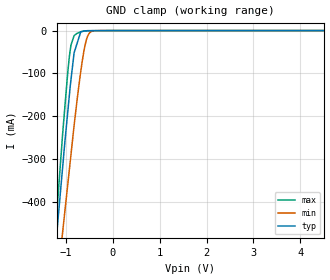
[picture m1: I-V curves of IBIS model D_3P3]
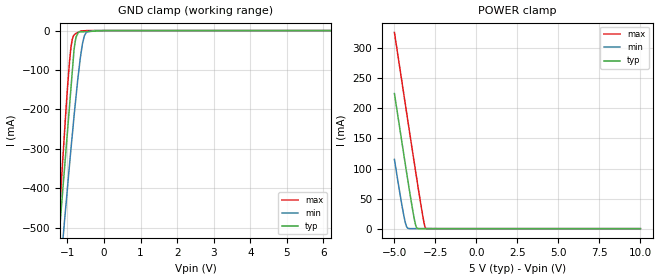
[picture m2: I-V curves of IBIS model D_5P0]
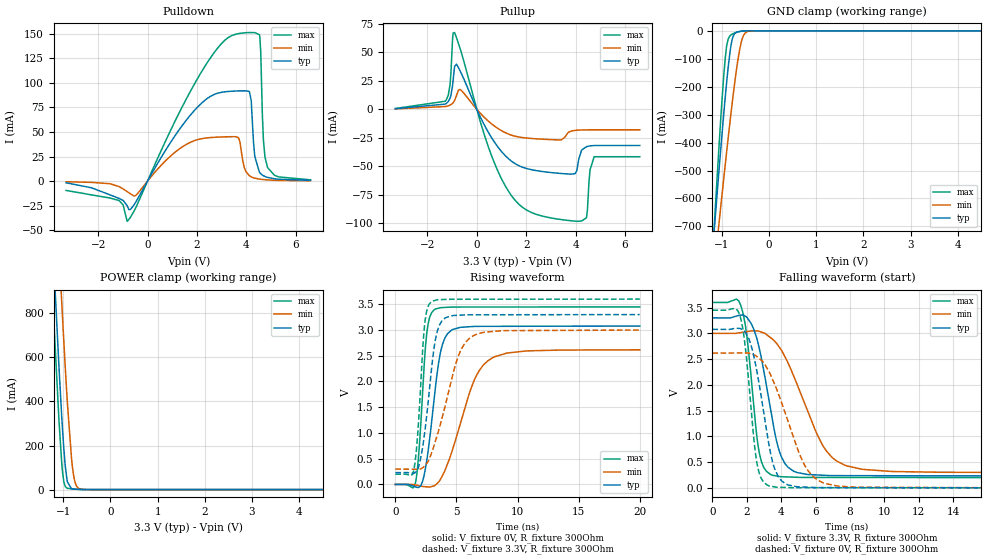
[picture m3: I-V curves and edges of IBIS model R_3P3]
|Texas Instruments Incorporated
|THVD14xx 3.3-V to 5V RS-485 Transceivers With +/-16kV IEC ESD Protection
[IBIS Ver]   4.1
[File name]   thvd1451.ibs
[File Rev]   1.0
[Date]   01/25/2018
[Source]
| Texas Instruments Incorporated.
| Analog-eLab Design Center, HPA
| 12500 TI Blvd
| Dallas, TX -75243
[Notes]   Revision History:
| Rev 1.0: 01/25/2018
| - Initial version of the model
| - Model generated from simulations in SPECTRE
| - Warnings regarding combined Non-monotonicity of various models have been
|   reviewed and considered minor and can be ignored.
| - Model names with a trailing _3P3 contain the model for
|   3.3V operation. Model names with a trailing _5P0 contain the model
|   for 5.0V operation.
| - C_comp although listed in numerical order of value are
|   obtained from varying PVT conditions. For PVT conditions for
|   each specific value refer the buffer description under
|   respective [Model]. IBIS model user is responsible for using
|   appropriate C_comp to simulate for Signal Integrity.
[Disclaimer]
| This model is designed as an aid for customers of Texas Instruments.
| TI and its licensors and suppliers make no warranties, either expressed
| or implied, with respect to this  model, including the warranties of
| merchantability or fitness for a particular purpose. The model is
| provided solely on an "as is" basis. The entire risk as to its quality
| and performance is with the customer.
| This model is subject to change without notice. Texas Instruments
| Incorporated is not responsible for updating this model.
[Copyright]
(C) Copyright 2018 Texas Instruments Incorporated.All rights reserved.
|  Component THVD1451DRB 8-pin VSON - DRB package
|  Part # THVD1451DRB
[Component]   THVD1451DRB
[Manufacturer]   TI
[Package]   |8 VSON - DRB package
|   typ   min   max
R_pkg   0.1   0.08   0.12
L_pkg   1.0nH   0.8nH   1.2nH
C_pkg   0.2pF   0.16pF   0.24pF
[Pin]   signal_name   model_name   R_pin   L_pin   C_pin
1   VCC   power   NA   NA   NA
2   R   R_OUTPUT   NA   NA   NA
3   D   D_INPUT   NA   NA   NA
4   GND   gnd   NA   NA   NA
5   Y   Y_OUTPUT   NA   NA   NA
6   Z   Z_OUTPUT   NA   NA   NA
7   B   nc   NA   NA   NA
8   A   nc   NA   NA   NA
[Diff Pin]  inv_pin  vdiff  tdelay_typ tdelay_min tdelay_max
5   6   2   NA   NA   NA
|   Model Selectors
[Model Selector]   R_OUTPUT
R_3P3   3.3V   3-state
R_5P0   5V   3-state
[Model Selector]   D_INPUT
D_3P3   3.3V   Input
D_5P0   5V   Input
[Model Selector]   Y_OUTPUT
Y_3P3   3.3V   3-state
Y_5P0   5V   3-state
[Model Selector]   Z_OUTPUT
Z_3P3   3.3V   3-state
Z_5P0   5V   3-state
| Models and submodels in the file (8): D_3P3 (Input), D_5P0 (Input), R_3P3 (3-state), R_5P0 (3-state), Y_3P3 (3-state), Y_5P0 (3-state), Z_3P3 (3-state), Z_5P0 (3-state)
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|   D_3P3 Model
[Model]   D_3P3
Model_type   Input
Vinl = 0.462
Vinh = 2.211
|   typ   min   max
C_comp   5.008pF   4.849pF   5.22pF
|  Where Nom  PVT is Nominal Process,   3.3V,  25C
|   Fast PVT is Strong Process,   3.6V, -40C
|   Slow PVT is Weak Process,   3V, 150C
[Model spec]
|subparameter
Vinl   0.462   0.420   0.504
Vinh   2.211   2.010   2.412
[Voltage Range]   3.3   3   3.6
|Junction Temperature
[Temperature Range]   25   150   -40
[Power Clamp Reference]   3.3   3   3.6
[GND Clamp Reference]   0   0   0
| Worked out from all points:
|   GND clamp passes 1 mA (typ) near -0.61 V on its own axis
[GND Clamp]
|   Voltage   I(typ)   I(min)   I(max)
-3.3V     -3.278A    -2.936A    -3.779A
-1.238V   -530.4mA   -649.5mA   -490.8mA
-1.189V   -467.6mA   -596.9mA   -418.7mA
-1.068V   -317.5mA   -469.6mA   -239.2mA
-923.8mV  -148.5mA   -322.6mA   -58.66mA
-892.5mV  -115.5mA   -290.6mA   -33.98mA
-825mV    -51.81mA   -221.8mA   -11.87mA
-686.9mV  -4.238mA   -98.87mA   -2.883mA
-611.5mV  -1.098mA   -45.16mA   -956uA
-556.5mV  -575.4uA   -19.03mA   -378.2uA
-389mV    -402.6uA   -378.7uA   -9.01uA
6.6V      0A         0A         0A
[POWER Clamp]
|   Voltage   I(typ)   I(min)   I(max)
-3.3V     0A         0A         0A
0V        0A         0A         0A
6.6V      0A         0A         0A
|   D_5p0 Model
[Model]   D_5P0
Model_type   Input
Vinl = 0.7
Vinh = 3.35
|   typ   min   max
C_comp   4.695pF   4.504pF   4.916pF
|  Where Nom  PVT is Nominal Process,   3.3V,  25C
|   Fast PVT is Strong Process,   3.6V, -40C
|   Slow PVT is Weak Process,   3V, 150C
[Model spec]
|subparameter
Vinl   0.462   0.420   0.504
Vinh   2.211   2.010   2.412
[Voltage Range]   5   4.5   5.5
|Junction Temperature
[Temperature Range]   25   150   -40
[Power Clamp Reference]   5   4.5   5.5
[GND Clamp Reference]   0   0   0
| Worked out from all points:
|   GND clamp passes 1 mA (typ) near -0.19 V on its own axis
|   POWER clamp passes 1 mA (typ) near -3.63 V on its own axis
[GND Clamp]
|   Voltage   I(typ)   I(min)   I(max)
-5V       -5.578A    -4.854A    -6.528A
-1.25V    -544.9mA   -660.5mA   -508.9mA
-1.141V   -419.4mA   -546.7mA   -345.5mA
-1.056V   -321.4mA   -458mA     -222.9mA
-991.4mV  -246.3mA   -389.9mA   -135.3mA
-905.3mV  -146.8mA   -301.1mA   -42.91mA
-819.4mV  -47.51mA   -216.6mA   -11.16mA
-790.6mV  -28.56mA   -189.8mA   -8.658mA
-642.3mV  -3.434mA   -65.57mA   -1.535mA
-539.2mV  -2.883mA   -13.61mA   -445uA
-274.1mV  -1.467mA   -25.44uA   -5.56uA
10V       0A         0A         0A
[POWER Clamp]
|   Voltage   I(typ)   I(min)   I(max)
-5V       224.6mA    115.1mA    326.4mA
-4.551V   145mA      40.18mA    245.7mA
-4.379V   114.6mA    15.3mA     214.9mA
-4.266V   94.83mA    3.843mA    194.5mA
-4.152V   75.1mA     313.8uA    174mA
-3.873V   28.68mA    17.01uA    124.3mA
-3.689V   4.175mA    15.82uA    91.91mA
-3.613V   505.7uA    15.33uA    78.66mA
-3.277V   23.7uA     13.15uA    22.02mA
-3.164V   22.37uA    12.42uA    6.07mA
-3.092V   21.53uA    11.95uA    735.4uA
10V       0A         0A         0A
|   R_3P3 Model
[Model]   R_3P3
Model_type   3-state
Polarity   Non-Inverting
Vmeas = 1.65
Vref = 0
Cref = 15pF
Rref = 100000
|   typ   min   max
C_comp   7.272pF   7.106pF   7.475pF
|  Where Nom  PVT is Nominal Process,   3.3V,  25C
|   Fast PVT is Strong Process,   3.6V, -40C
|   Slow PVT is Weak Process,   3V, 150C
[Voltage Range]   3.3   3   3.6
|Junction Temperature
[Temperature Range]   25   150   -40
[Pullup Reference]   3.3   3   3.6
[Pulldown Reference]   0   0   -0
[Power Clamp Reference]   3.3   3   3.6
[GND Clamp Reference]   0   0   0
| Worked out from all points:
|   slope of the pulldown table from 0 to 0.495 V, typ, clamps not added: 22.9 ohm
|   slope of the pullup table from 0 to 0.495 V, typ, clamps not added: 23.3 ohm
|   GND clamp passes 1 mA (typ) near -0.56 V on its own axis
|   POWER clamp passes 1 mA (typ) near -0.67 V on its own axis
|   falling waveform, V_fixture 3.3V, R_fixture 300Ohm: 20-80 % time 1.04ns typ, 2.04ns min, 619ps max; typ from 3.3 V to 0.23 V
|   rising waveform, V_fixture 0V, R_fixture 300Ohm: 20-80 % time 951ps typ, 2.12ns min, 551ps max; typ from 0 V to 3.08 V
|   rising waveform, V_fixture 3.3V, R_fixture 300Ohm: 20-80 % time 883ps typ, 1.83ns min, 528ps max; typ from 0.23 V to 3.3 V
|   falling waveform, V_fixture 0V, R_fixture 300Ohm: 20-80 % time 953ps typ, 1.73ns min, 594ps max; typ from 3.08 V to 0 V
[Pulldown]
|   Voltage   I(typ)   I(min)   I(max)
-3.3V     -1.729mA   -655.1uA   -9.49mA
-1.147V   -17.66mA   -5.603mA   -19.81mA
-824.9mV  -24.97mA   -10.66mA   -40.91mA
2.339V    82.53mA    43.75mA    117.4mA
3.666V    91.77mA    44.44mA    150mA
4.123V    91.25mA    5.492mA    151.2mA
4.2V      82.07mA    4.323mA    151.1mA
4.344V    25.07mA    3.001mA    151.1mA
4.549V    8.499mA    2.003mA    147mA
4.694V    5.479mA    1.577mA    41.97mA
4.862V    3.775mA    1.232mA    13.8mA
6.6V      725.2uA    297.7uA    1.276mA
[GND Clamp]
|   Voltage   I(typ)   I(min)   I(max)
-3.3V     -5.574A    -4.524A    -7.37A
-1.176V   -743.8mA   -877.1mA   -741.4mA
-1.125V   -633.4mA   -792.5mA   -591.8mA
-1.063V   -504.9mA   -693.2mA   -420.1mA
-926.2mV  -232.9mA   -475.2mA   -93.33mA
-895.8mV  -178.7mA   -428.3mA   -51.39mA
-824.9mV  -72.33mA   -321.6mA   -17.07mA
-731.1mV  -10.51mA   -190mA     -7.947mA
-662mV    -3.564mA   -106mA     -4.061mA
-568.5mV  -1.111mA   -28.27mA   -1.242mA
-400.8mV  -67.49uA   -653.7uA   -47.19uA
6.6V      0A         0A         0A
[Pullup]
|   Voltage   I(typ)   I(min)   I(max)
-3.3V     560.1uA    370.5uA    728.3uA
-1.278V   4.569mA    2.429mA    7.078mA
-1.085V   9.719mA    3.69mA     21.67mA
-899.7mV  37.67mA    7.766mA    67.27mA
588.8mV   -24.59mA   -12.6mA    -40.21mA
1.861V    -50.84mA   -24.8mA    -86.1mA
3.982V    -56.41mA   -18.45mA   -98.02mA
4.244V    -35.68mA   -18.11mA   -97.86mA
4.442V    -32.74mA   -18.02mA   -95.02mA
4.585V    -32.09mA   -17.98mA   -53.08mA
4.754V    -31.72mA   -17.96mA   -41.54mA
6.6V      -31.72mA   -17.96mA   -41.54mA
[POWER Clamp]
|   Voltage   I(typ)   I(min)   I(max)
-3.3V     11.22A     11.71A     11A
-1.249V   1.241A     1.795A     985.5mA
-1.198V   1.016A     1.569A     760.7mA
-1.09V    553.2mA    1.093A     310.5mA
-1.032V   328.7mA    847.9mA    118.7mA
-987.6mV  184.1mA    670.5mA    34.96mA
-917.6mV  39.86mA    410.4mA    6.101mA
-824.9mV  3.812mA    142mA      3.29mA
-784.8mV  2.338mA    70.64mA    2.65mA
-719.5mV  1.432mA    16.69mA    1.743mA
-629.9mV  696.7uA    2.159mA    783.2uA
6.6V      0A         0A         0A
[Ramp]
R_load = 300
|   typ   min   max
dV/dt_r   1.84616/9.47025e-10   1.56867/2.11704e-09   2.06964/5.49202e-10
dV/dt_f   1.84214/1.03769e-09   1.62061/2.04134e-09   2.04095/6.18768e-10
[Falling Waveform]
V_fixture = 3.3V
V_fixture_min = 3V
V_fixture_max = 3.6V
R_fixture = 300Ohm
C_fixture = 0F
|   Time   V(typ)   V(min)   V(max)
0s        3.3V       2.999V     3.6V
1.66ns    3.354V     3.015V     3.527V
2.011ns   3.306V     3.033V     2.916V
2.7ns     2.741V     3.041V     725.1mV
3.363ns   1.561V     2.92V      263.3mV
3.865ns   738.8mV    2.743V     222.7mV
4.41ns    395.4mV    2.415V     211.4mV
6.35ns    246.5mV    862.6mV    202.3mV
7.629ns   237.1mV    450.3mV    201.9mV
20ns      229.6mV    298.3mV    198.4mV
[Rising Waveform]
V_fixture = 0V
V_fixture_min = 0V
V_fixture_max = 0V
R_fixture = 300Ohm
C_fixture = 0F
|   Time   V(typ)   V(min)   V(max)
0s        266.4uV    702.8uV    62.26uV
1.638ns   -44.93mV   -10.88mV   25.31mV
1.942ns   -52.48mV   -25.47mV   674.8mV
2.548ns   430.2mV    -46.59mV   2.888V
3.175ns   1.662V     -26.29mV   3.392V
3.704ns   2.578V     105.8mV    3.435V
4.28ns    2.93V      406.6mV    3.442V
6.471ns   3.07V      2.034V     3.447V
7.918ns   3.072V     2.456V     3.447V
20ns      3.077V     2.615V     3.449V
[Rising Waveform]
V_fixture = 3.3V
V_fixture_min = 3V
V_fixture_max = 3.6V
R_fixture = 300Ohm
C_fixture = 0F
|   Time   V(typ)   V(min)   V(max)
0s        229.6mV    298.3mV    198.4mV
1.496ns   213.8mV    294.8mV    263mV
1.837ns   300.7mV    294mV      1.003V
2.389ns   985.7mV    356.7mV    3.089V
2.942ns   2.202V     597.7mV    3.55V
3.325ns   2.868V     879.5mV    3.581V
3.803ns   3.174V     1.276V     3.592V
5.173ns   3.287V     2.505V     3.597V
6.35ns    3.295V     2.885V     3.598V
20ns      3.3V       2.999V     3.6V
[Falling Waveform]
|Gnd
V_fixture = 0V
V_fixture_min = 0V
V_fixture_max = 0V
R_fixture = 300Ohm
C_fixture = 0F
|   Time   V(typ)   V(min)   V(max)
0s        3.077V     2.615V     3.449V
1.592ns   3.095V     2.619V     3.349V
1.925ns   3.014V     2.62V      2.691V
2.568ns   2.29V      2.553V     517.6mV
3.175ns   1.059V     2.322V     56.64mV
3.554ns   437.2mV    2.06V      22.68mV
4.059ns   124.3mV    1.619V     9.922mV
5.313ns   14.91mV    471.6mV    3.698mV
6.413ns   5.424mV    101.2mV    3.426mV
20ns      266.3uV    702.7uV    61.95uV
